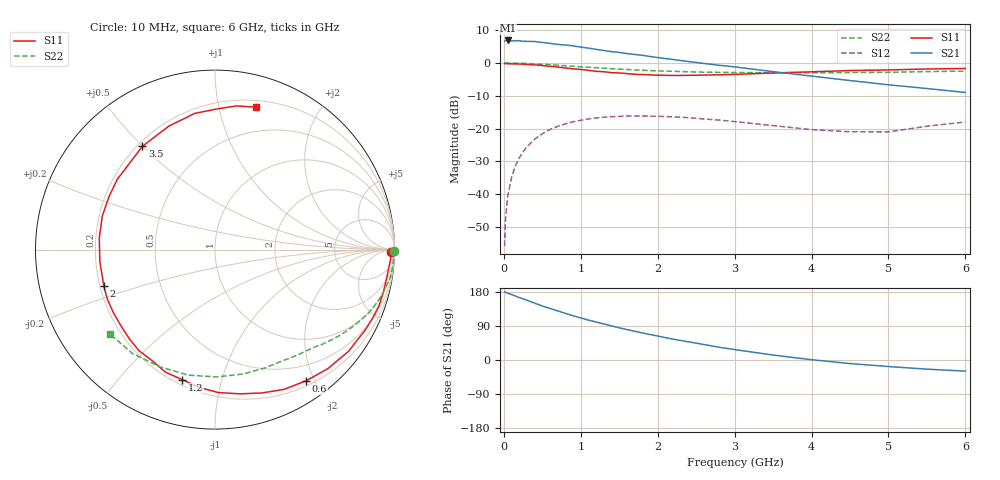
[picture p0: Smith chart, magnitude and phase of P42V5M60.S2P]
! SIEMENS Small Signal Semiconductors
! BFP182
! Si NPN RF Bipolar Junction Transistor in SOT143
! VCE = 2.5 V  IC = 0.6 mA
! Common Emitter S-Parameters:  March  1996
# GHz  S  MA  R  50
!  f  S11  S21  S12  S22
! GHz  MAG  ANG  MAG  ANG  MAG  ANG  MAG  ANG
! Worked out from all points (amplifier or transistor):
!   36 points, 10 MHz to 6 GHz, reference 50 ohm
!   highest |S21| = 6.9 dB at 50 MHz (marker M1)
!   |S21| within 3 dB of that: start of sweep to 1.282 GHz
!   unconditionally stable (mu >= 1): 2.855 GHz to end of sweep
!   at 250 MHz: K = 0.09, MSG = 16.9 dB, |S12| = -27.1 dB
!   at 1.4 GHz: K = 0.50, MSG = 9.9 dB, |S12| = -16.4 dB
!   at 6 GHz: K = 1.20, MAG = 1.8 dB, |S12| = -18.0 dB
!   S11 on the Smith chart (normalised r, x): 10 MHz: 60, -43; 600 MHz: 0.27, -1.88; 1.2 GHz: 0.23, -0.75; 2 GHz: 0.22, -0.15; 3.5 GHz: 0.22, +0.50; 6 GHz: 0.26, +1.29
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0.01  0.9783 -0.9  2.171 179.6  0.0016 88.6  0.999 -0.3
0.02  0.9824 -2.0  2.192 179.2  0.0038 87.9  0.9961 -0.6
0.05  0.9762 -4.7  2.209 176.3  0.0093 88.5  0.9983 -1.7
0.1  0.9694 -9.3  2.17 172.6  0.0178 83.8  0.9956 -3.4
0.15  0.9676 -14.1  2.184 168.8  0.027 81.0  0.995 -5.2
0.2  0.966 -18.8  2.195 164.8  0.0356 78.1  0.9917 -6.9
0.25  0.9582 -23.2  2.142 161.2  0.0442 75.1  0.989 -8.7
0.4  0.9356 -37.2  2.129 149.9  0.0686 65.8  0.9709 -13.4
0.6  0.8899 -55.2  1.996 136.1  0.0967 54.8  0.942 -19.5
0.9  0.8153 -80.3  1.827 116.8  0.1268 39.7  0.8918 -27.3
1.1  0.7721 -96.7  1.689 105.3  0.14 31.3  0.8605 -31.9
1.2  0.7472 -104.2  1.613 100.2  0.1451 26.9  0.847 -34.1
1.6  0.6888 -133.9  1.393 80.3  0.1556 13.7  0.7981 -41.4
2  0.652 -161.7  1.21 63.2  0.1538 3.4  0.758 -48.2
2.2  0.6451 -174.1  1.132 55.0  0.1506 -1.2  0.7466 -51.8
2.8  0.6601 153.5  0.923 33.7  0.1345 -11.0  0.7188 -62.6
3.5  0.7033 125.1  0.738 13.1  0.1108 -15.5  0.7107 -77.3
4  0.734 110.6  0.631 0.8  0.0962 -11.8  0.7095 -89.2
4.5  0.7672 98.5  0.54 -9.4  0.0892 -4.5  0.7151 -102.0
5  0.7837 89.2  0.465 -17.2  0.089 8.6  0.7215 -115.0
5.5  0.8098 81.4  0.408 -24.2  0.1083 14.0  0.7391 -128.5
6  0.8249 74.1  0.355 -29.3  0.1259 14.9  0.7518 -141.4
